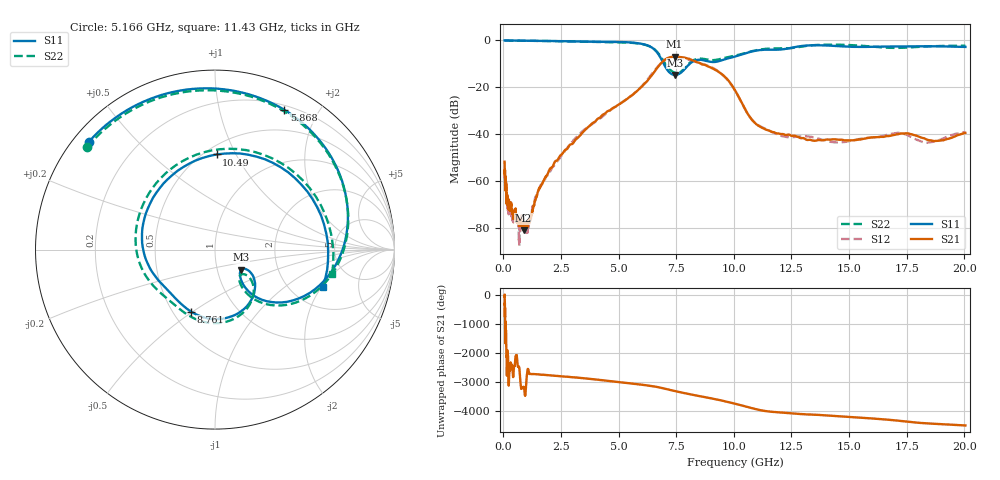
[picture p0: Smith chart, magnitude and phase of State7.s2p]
# Hz S DB R 50
!freq MagS11 AngS11 MagS21 AngS21 MagS12 AngS12 MagS22 AngS22
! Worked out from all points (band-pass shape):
!   1601 points, 50 MHz to 20.05 GHz, reference 50 ohm
!   highest |S21| = -6.91 dB at 7.43 GHz (marker M1); lowest = -81.1 dB at 871.7 MHz (marker M2)
!   |S21| within 3 dB of the highest: 6.822 GHz to 8.565 GHz (1.743 GHz wide, 22.7 % of centre)
!   lowest |S11| = -14.7 dB at 7.458 GHz (marker M3), VSWR 1.45, Z = 65 - j15.2 ohm
!   |S11| at or under -10 dB: 6.959 GHz to 8.083 GHz (1.124 GHz wide, 15 % of centre)
!   |S22| runs from -13.9 to 0.0 dB; largest |S21 - S12| = 0.023
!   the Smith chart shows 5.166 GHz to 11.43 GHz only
!   S11 on the Smith chart (normalised r, x): 5.166 GHz: 0.04, +0.37; 5.868 GHz: 0.25, +1.59; 8.761 GHz: 0.61, -0.49; 10.49 GHz: 0.57, +0.84; 11.43 GHz: 2.96, -2.04
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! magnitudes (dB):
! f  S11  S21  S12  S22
! 50 MHz  0.0  -51.8  -57.0  0.0
! 87.7 MHz  0.0  -61.5  -63.1  0.0
! 99.62 MHz  0.0  -63.8  -59.3  0.0
! 135.9 MHz  0.0  -65.1  -66.5  0.0
! 213.9 MHz  0.0  -69.8  -72.5  0.0
! 369.6 MHz  0.0  -73.1  -74.4  0.0
! 680.7 MHz  -0.1  -77.5  -86.2  -0.1
! 871.7 MHz  -0.1  -81.1  -76.8  -0.1
! 1.005 GHz  -0.1  -79.3  -81.5  -0.1
! 2.722 GHz  -0.3  -46.6  -46.5  -0.4
! 5.166 GHz  -0.7  -26.3  -26.2  -0.8
! 5.868 GHz  -1.2  -20.9  -20.9  -1.3
! 6.517 GHz  -3.6  -13.8  -13.3  -3.5
! 7.402 GHz  -14.7  -6.9  -7.2  -13.7
! 7.43 GHz  -14.7  -6.9  -7.1  -13.8
! 7.458 GHz  -14.7  -6.9  -7.2  -13.9
! 8.761 GHz  -8.6  -10.5  -10.4  -8.0
! 9.657 GHz  -7.9  -16.0  -16.1  -7.3
! 10.49 GHz  -5.5  -29.3  -29.4  -5.4
! 11.43 GHz  -3.9  -38.2  -38.0  -3.5
! 14.53 GHz  -2.4  -42.4  -43.6  -1.8
! 20.05 GHz  -2.8  -39.5  -39.1  -2.2
